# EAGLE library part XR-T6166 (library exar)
Codirectional digital PROCESSOR
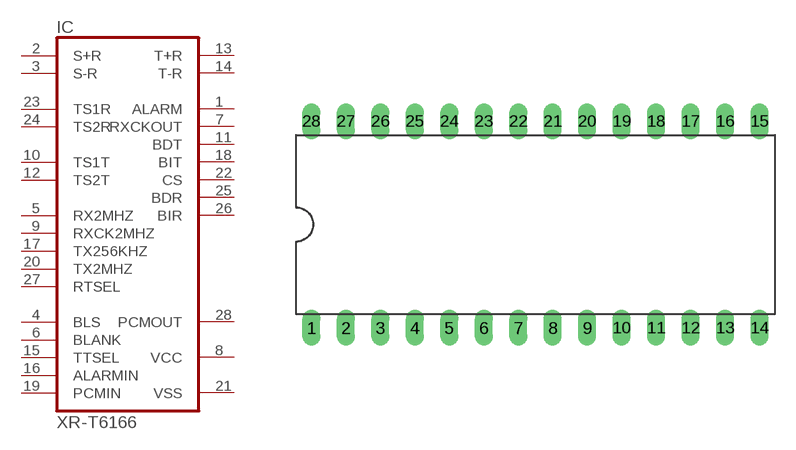
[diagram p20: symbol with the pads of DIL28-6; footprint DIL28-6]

Designator prefix IC

## XR-T6166 (OC_FARNELL: unknown; OC_NEWARK: unknown)  [DIL28-6]
1  ALARM  out
2  S+R  in
3  S-R  in
4  BLS  in
5  RX2MHZ  in
6  BLANK  in
7  RXCKOUT  out
8  VCC  pwr
9  RXCK2MHZ  in
10  TS1T  in
11  BDT  out
12  TS2T  in
13  T+R  out
14  T-R  out
15  TTSEL  in
16  ALARMIN  in
17  TX256KHZ  in
18  BIT  out
19  PCMIN  in
20  TX2MHZ  in
21  VSS  pwr
22  CS  out
23  TS1R  in
24  TS2R  in
25  BDR  out
26  BIR  out
27  RTSEL  in
28  PCMOUT  out

## Footprint DIL28-6 (pad centres in mm)
Dual In Line Package 0.6 inch
drill 0.813 long: 1 -16.51,-7.62; 2 -13.97,-7.62; 3 -11.43,-7.62; 4 -8.89,-7.62; 5 -6.35,-7.62; 6 -3.81,-7.62; 7 -1.27,-7.62; 8 1.27,-7.62; 9 3.81,-7.62; 10 6.35,-7.62; 11 8.89,-7.62; 12 11.43,-7.62; 13 13.97,-7.62; 14 16.51,-7.62; 15 16.51,7.62; 16 13.97,7.62; 17 11.43,7.62; 18 8.89,7.62; 19 6.35,7.62; 20 3.81,7.62; 21 1.27,7.62; 22 -1.27,7.62; 23 -3.81,7.62; 24 -6.35,7.62; 25 -8.89,7.62; 26 -11.43,7.62; 27 -13.97,7.62; 28 -16.51,7.62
